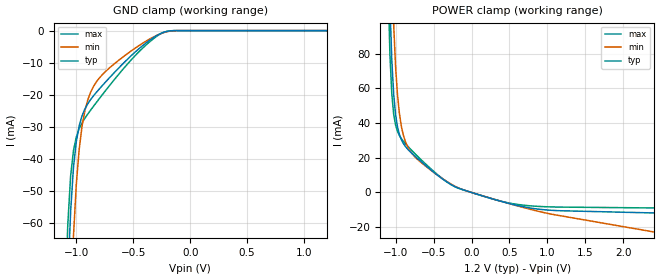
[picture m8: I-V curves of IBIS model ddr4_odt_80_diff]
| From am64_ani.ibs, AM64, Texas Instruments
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|   Model ddr4_odt_80_diff
[Model] ddr4_odt_80_diff
Model_type Input
Polarity   Non-Inverting
Enable   Active-High
Vinl =  0.700V
Vinh =  0.900V
C_comp   2.664pF   2.643pF   2.684pF
[Model Spec]
Vinh   0.900V   0.820V   0.980V
Vinl   0.700V   0.620V   0.780V
[Temperature Range]   25.000   0.125k   -40.000
[Voltage Range]   1.200V   1.140V   1.260V
[C Comp Corner]
C_comp   2.643pF   2.664pF   2.684pF
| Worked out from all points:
|   GND clamp passes 1 mA (typ) near -0.26 V on its own axis
|   POWER clamp passes 1 mA (typ) near -0.07 V on its own axis
[GND_clamp]
|Voltage   I(typ)   I(min)   I(max)
-1.2V     -390mA     -438.6mA   -365.5mA
-1.075V   -79.16mA   -120mA     -60.71mA
-1.05V    -56.54mA   -87.53mA   -45.42mA
-1.025V   -42.79mA   -64.14mA   -37.47mA
-1V       -34.66mA   -47.99mA   -33.19mA
-975mV    -29.76mA   -37.14mA   -30.62mA
-950mV    -26.65mA   -29.91mA   -28.82mA
-875mV    -21.56mA   -19.3mA    -24.86mA
-775mV    -17.29mA   -13.88mA   -20.18mA
-550mV    -8.918mA   -7.167mA   -10.41mA
-200mV    -203.5uA   -308.6uA   -187.4uA
1.2V      0A         0A         0A
[POWER_clamp]
|Voltage   I(typ)   I(min)   I(max)
-1.2V     597.6mA    736.4mA    625.3mA
-1.1V     160.8mA    252.2mA    123.7mA
-1.075V   109.3mA    183mA      80.02mA
-1.05V    76.4mA     132.2mA    56.93mA
-1.025V   56.58mA    96.67mA    45.15mA
-1V       44.9mA     72.5mA     38.91mA
-975mV    37.91mA    56.37mA    35.26mA
-925mV    30.57mA    38.44mA    31.1mA
-825mV    24.28mA    25.1mA     26mA
-300mV    5.383mA    5.65mA     5.398mA
825mV     -9.3mA     -10.27mA   -7.873mA
2.4V      -11.82mA   -22.76mA   -8.928mA
